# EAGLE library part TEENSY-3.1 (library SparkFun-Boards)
Teensy 3+ Footprint Mechanical footprint with connectors for Teensy Development Board with ARM Cortex. SparkFun Products: Teensy 3.2 Teensy LC
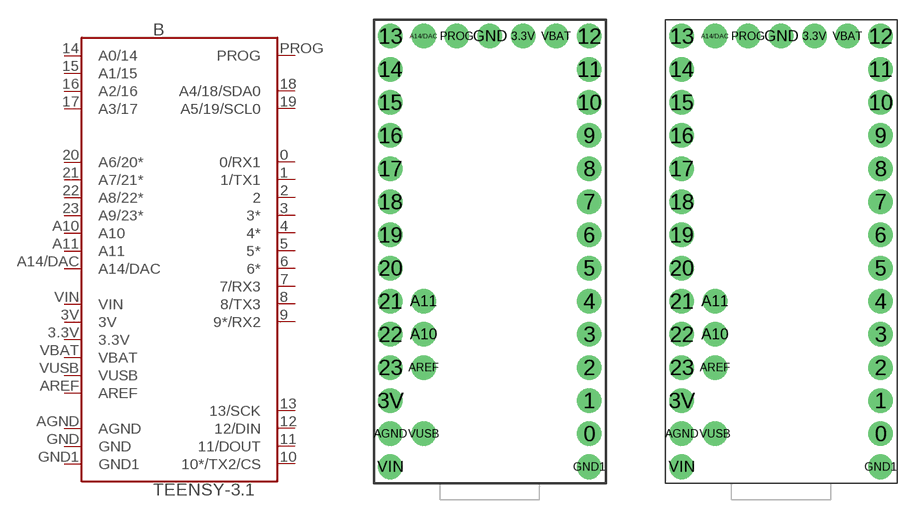
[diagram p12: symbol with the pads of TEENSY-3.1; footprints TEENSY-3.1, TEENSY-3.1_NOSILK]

Designator prefix B

## TEENSY-3.1SILK (SF_ID: DEV-12646)  [TEENSY-3.1]
0  0/RX1
1  1/TX1
2  2
3  3*
3.3V  3.3V  pwr
3V  3V  pwr
4  4*
5  5*
6  6*
7  7/RX3
8  8/TX3
9  9*/RX2
10  10*/TX2/CS
11  11/DOUT
12  12/DIN
13  13/SCK
14  A0/14
15  A1/15
16  A2/16
17  A3/17
18  A4/18/SDA0
19  A5/19/SCL0
20  A6/20*
21  A7/21*
22  A8/22*
23  A9/23*
A10  A10
A11  A11
A14/DAC  A14/DAC
AGND  AGND  pwr
AREF  AREF
GND  GND  pwr
GND1  GND1  pwr
PROG  PROG
VBAT  VBAT  pwr
VIN  VIN  pwr
VUSB  VUSB  pwr

## TEENSY-3.1NOSILK (SF_ID: DEV-12646)  [TEENSY-3.1_NOSILK]
Pads as for TEENSY-3.1

## Footprint TEENSY-3.1 (pad centres in mm)
Teensy 3 Footprint Specifications: Pin count:37 Pin pitch: 0.1" Area:0.7x1.4" Example device(s): Teensy 3.1
drill 1.016 pad 1.88: 0 7.62,-13.97; 1 7.62,-11.43; 2 7.62,-8.89; 3 7.62,-6.35; 3.3V 2.54,16.51; 3V -7.62,-11.43; 4 7.62,-3.81; 5 7.62,-1.27; 6 7.62,1.27; 7 7.62,3.81; 8 7.62,6.35; 9 7.62,8.89; 10 7.62,11.43; 11 7.62,13.97; 12 7.62,16.51; 13 -7.62,16.51; 14 -7.62,13.97; 15 -7.62,11.43; 16 -7.62,8.89; 17 -7.62,6.35; 18 -7.62,3.81; 19 -7.62,1.27; 20 -7.62,-1.27; 21 -7.62,-3.81; 22 -7.62,-6.35; 23 -7.62,-8.89; A10 -5.08,-6.35; A11 -5.08,-3.81; A14/DAC -5.08,16.51; AGND -7.62,-13.97; AREF -5.08,-8.89; GND 0,16.51; GND1 7.62,-16.51; PROG -2.54,16.51; VBAT 5.08,16.51; VIN -7.62,-16.51; VUSB -5.08,-13.97

## Footprint TEENSY-3.1_NOSILK (pad centres in mm)
Teensy 3 Footprint- No Silk Label on Pins Specifications: Pin count:37 Pin pitch: 0.1" Area:0.7x1.4" Example device(s): Teensy 3.1
drill 1.016 pad 1.88: 0 7.62,-13.97; 1 7.62,-11.43; 2 7.62,-8.89; 3 7.62,-6.35; 3.3V 2.54,16.51; 3V -7.62,-11.43; 4 7.62,-3.81; 5 7.62,-1.27; 6 7.62,1.27; 7 7.62,3.81; 8 7.62,6.35; 9 7.62,8.89; 10 7.62,11.43; 11 7.62,13.97; 12 7.62,16.51; 13 -7.62,16.51; 14 -7.62,13.97; 15 -7.62,11.43; 16 -7.62,8.89; 17 -7.62,6.35; 18 -7.62,3.81; 19 -7.62,1.27; 20 -7.62,-1.27; 21 -7.62,-3.81; 22 -7.62,-6.35; 23 -7.62,-8.89; A10 -5.08,-6.35; A11 -5.08,-3.81; A14/DAC -5.08,16.51; AGND -7.62,-13.97; AREF -5.08,-8.89; GND 0,16.51; GND1 7.62,-16.51; PROG -2.54,16.51; VBAT 5.08,16.51; VIN -7.62,-16.51; VUSB -5.08,-13.97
